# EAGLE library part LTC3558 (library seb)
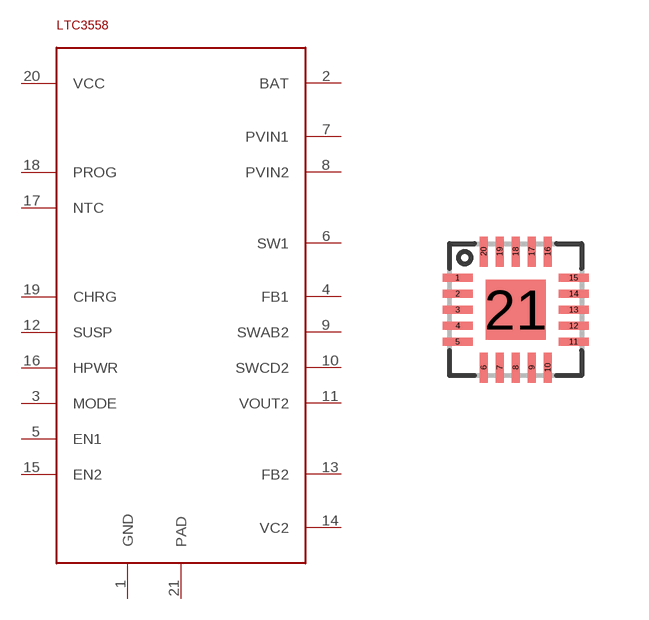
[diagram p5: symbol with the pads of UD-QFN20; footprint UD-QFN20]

Designator prefix IC

## LTC3558  [UD-QFN20]
1  GND
2  BAT
3  MODE
4  FB1
5  EN1
6  SW1
7  PVIN1
8  PVIN2
9  SWAB2
10  SWCD2
11  VOUT2
12  SUSP
13  FB2
14  VC2
15  EN2
16  HPWR
17  NTC
18  PROG
19  CHRG
20  VCC
21  PAD

## Footprint UD-QFN20 (pad centres in mm)
smd 0.751 x 0.2: 1 -1.451,0.8; 2 -1.451,0.4; 3 -1.451,0; 4 -1.451,-0.4; 5 -1.451,-0.8; 11 1.451,-0.8; 12 1.451,-0.4; 13 1.451,0; 14 1.451,0.4; 15 1.451,0.8
smd 0.2 x 0.751: 6 -0.8,-1.451; 7 -0.4,-1.451; 8 0,-1.451; 9 0.4,-1.451; 10 0.8,-1.451; 16 0.8,1.451; 17 0.4,1.451; 18 0,1.451; 19 -0.4,1.451; 20 -0.8,1.451
smd 1.5 x 1.5: 21 0,0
